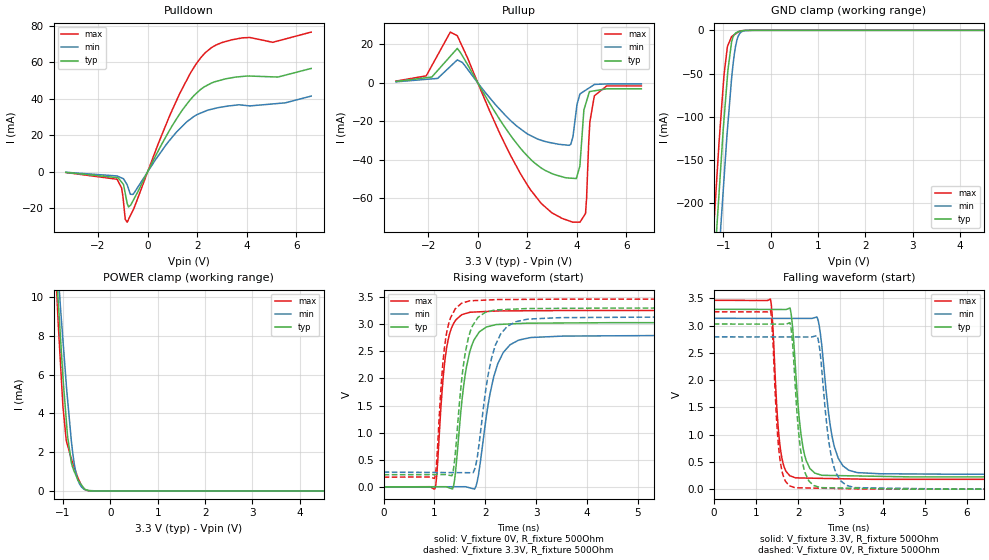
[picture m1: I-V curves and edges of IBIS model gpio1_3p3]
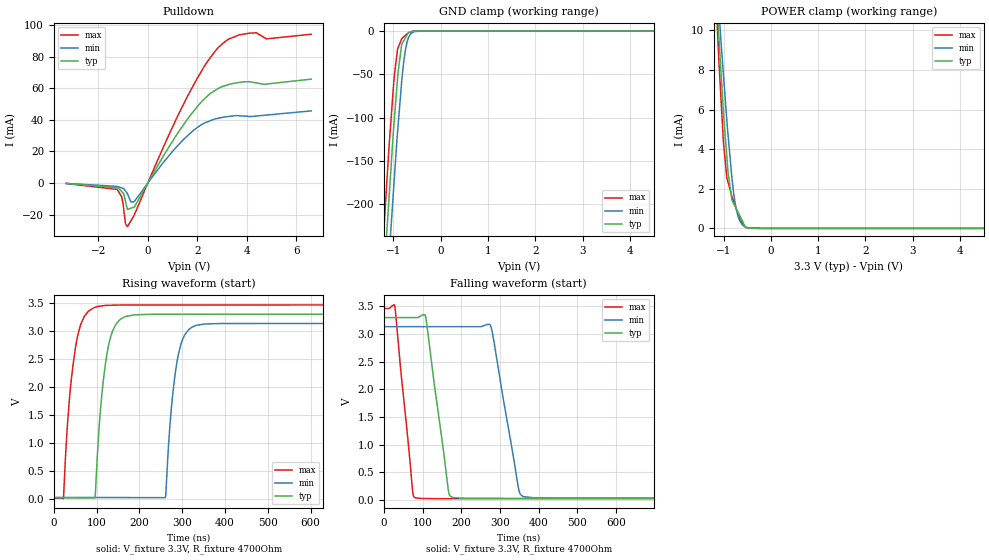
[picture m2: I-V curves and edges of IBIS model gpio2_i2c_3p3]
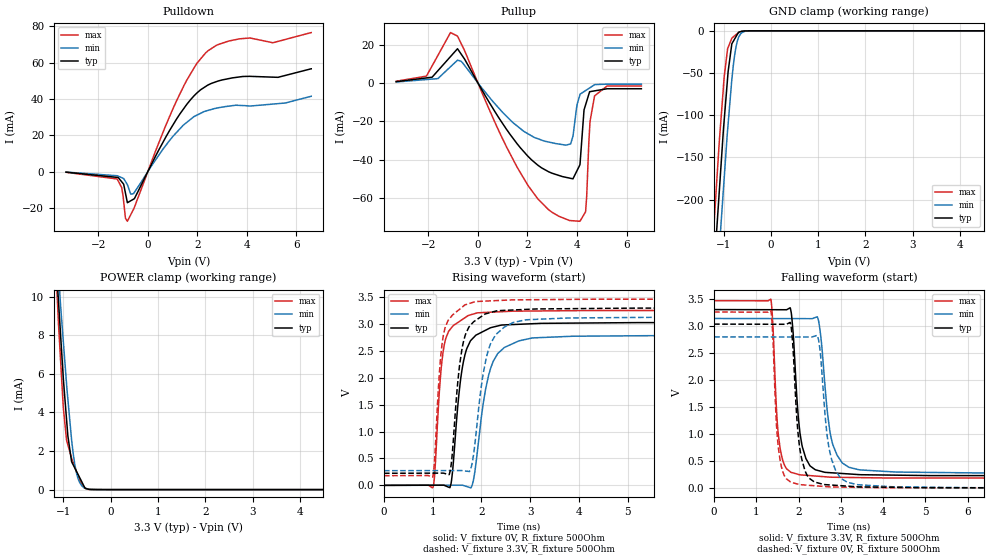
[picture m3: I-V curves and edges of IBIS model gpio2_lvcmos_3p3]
| Texas Instruments Incorporated
| CDCI6214
| Marketing part#   Digital Voltage Range   Package-type   #pins
| CDCI6214   1.71V - 3.465V   QFN   24
[IBIS Ver]   5.0
[File name]   cdci6214.ibs
[File Rev]   1.0
[Date]   10/26/2018
[Source]
| Texas Instruments Incorporated.
| Online Design Tools
| 12500 TI Blvd
| Dallas, TX -75243
[Notes]   Revision History:
| Rev 1.1: 10/26/2018
| - Pin1 and 2 name updated.
| Rev 1.0: 08/24/2017
| - Initial version of the model
| - Model generated from simulations in SPECTRE
| - Model matched to SPICE simulation
| - C_comp although listed in numerical order of value are
|   obtained from varying PVT conditions. For PVT conditions for
|   each specific value refer the buffer description under
|   respective [Model]. IBIS model user is responsible for using
|   appropriate C_comp to simulate for Signal Integrity.
| - Notes regarding combined Non-monotonicity of various models
|   have been reviewed and considered minor and can be ignored.
[Disclaimer]
| This model is designed as an aid for customers of Texas Instruments.
| TI and its licensors and suppliers make no warranties, either expressed
| or implied, with respect to this  model, including the warranties of
| merchantability or fitness for a particular purpose. The model is
| provided solely on an "as is" basis. The entire risk as to its quality
| and performance is with the customer.
[Copyright]
(C) Copyright 2017 Texas Instruments Incorporated.All rights reserved.
|   CDCI6214
[Component]   CDCI6214
[Manufacturer]   TI
[Package]   |24 QFN
|   typ   min   max
R_pkg   0.08328ohm   0.00805ohm   0.12644ohm
L_pkg   0.9771nH   0.25585nH   1.39654nH
C_pkg   0.1809pF   0.13118pF   0.62699pF
[Pin]   signal_name   model_name   R_pin   L_pin   C_pin
1   XOUT/FB   input1   0.00805ohm   0.25585nH   0.62699pF
2   XIN/FB   input2   0.08466ohm   0.93051nH   0.14630pF
3   VDD_REF   power   0.04341ohm   0.67199nH   0.16682pF
4   REF_SEL   input3   0.08490ohm   0.93218nH   0.14358pF
5   REFP   refp   0.08517ohm   0.93587nH   0.14543pF
6   REFN   refn   0.08525ohm   0.94279nH   0.13118pF
7   Y0   output   0.09517ohm   1.04961nH   0.13714pF
8   RESETN/SYNC   gpio1   0.08356ohm   0.91705nH   0.14348pF
9   Y4N   diff_out   0.08217ohm   0.90083nH   0.14310pF
10   Y4P   diff_out   0.09011ohm   0.98297nH   0.14845pF
11   OE/GPIO4   gpio1   0.08464ohm   0.92609nH   0.14498pF
12   SCL/GPIO3   input4   0.10102ohm   1.10915nH   0.14502pF
13   Y3N   diff_out   0.11209ohm   1.23284nH   0.15766pF
14   Y3P   diff_out   0.10303ohm   1.12457nH   0.16392pF
15   VDDO_34   power   0.03522ohm   0.70101nH   0.22084pF
16   VDDO_12   power   0.05257ohm   0.81073nH   0.20015pF
17   Y2N   diff_out   0.10909ohm   1.19284nH   0.16931pF
18   Y2P   diff_out   0.12644ohm   1.39654nH   0.16716pF
19   SDA/GPIO2   gpio2   0.05815ohm   0.96344nH   0.18512pF
20   STATUS/GPIO1   gpio1   0.10342ohm   1.13184nH   0.16054pF
21   Y1N   diff_out   0.10724ohm   1.17298nH   0.16355pF
22   Y1P   diff_out   0.10246ohm   1.12101nH   0.15895pF
23   EEPROMSEL   input3   0.10472ohm   1.14805nH   0.17052pF
24   VDD_VCO   power   0.05614ohm   0.89989nH   0.20226pF
[Diff Pin]   inv_pin   vdiff   tdelay_typ  tdelay_min  tdelay_max
5   6   200mV   NA   NA   NA
10   9   NA   NA   NA   NA
14   13   NA   NA   NA   NA
18   17   NA   NA   NA   NA
22   21   NA   NA   NA   NA
|   Model Selectors
[Model Selector] gpio1
gpio1_1p8   1.8V   I/O
gpio1_2p5   2.5V   I/O
gpio1_3p3   3.3V   I/O
[Model Selector] gpio2
gpio2_i2c_1p8   1.8V   I/O_open_drain
gpio2_i2c_2p5   2.5V   I/O_open_drain
gpio2_i2c_3p3   3.3V   I/O_open_drain
gpio2_lvcmos_1p8  1.8V   I/O
gpio2_lvcmos_2p5  2.5V   I/O
gpio2_lvcmos_3p3  3.3V   I/O
[Model Selector] input1
input1_1p8   1.8V   Input
input1_2p5   2.5V   Input
input1_3p3   3.3V   Input
[Model Selector] input2
input2_1p8   1.8V   Input
input2_2p5   2.5V   Input
input2_3p3   3.3V   Input
[Model Selector] input3
input3_1p8   1.8V   Input
input3_2p5   2.5V   Input
input3_3p3   3.3V   Input
[Model Selector] input4
input4_1p8   1.8V   Input
input4_2p5   2.5V   Input
input4_3p3   3.3V   Input
[Model Selector] output
output_fast_1p8   1.8V   3-state
output_fast_2p5   2.5V   3-state
output_fast_3p3   3.3V   3-state
output_slow_1p8   1.8V   3-state
output_slow_2p5   2.5V   3-state
output_slow_3p3   3.3V   3-state
[Model Selector] refn
refn_1p8   1.8V   Input
refn_2p5   2.5V   Input
refn_3p3   3.3V   Input
[Model Selector] refp
refp_1p8   1.8V   Input
refp_2p5   2.5V   Input
refp_3p3   3.3V   Input
[Model Selector] diff_out
cml_1p8   1.8V   3-state
cml_2p5   2.5V   3-state
cml_3p3   3.3V   3-state
hcsl_1p8   1.8V   Open_source
hcsl_2p5   2.5V   Open_source
hcsl_3p3   3.3V   Open_source
lvds_1p8   1.8V   3-state
lvds_2p5   2.5V   3-state
lvds_3p3   3.3V   3-state
lvpecl_1p8   1.8V   3-state
lvpecl_2p5   2.5V   3-state
lvpecl_3p3   3.3V   3-state
| Models and submodels in the file (45): gpio1_1p8 (I/O), gpio1_2p5 (I/O), gpio1_3p3 (I/O), gpio2_i2c_1p8 (I/O_open_drain), gpio2_i2c_2p5 (I/O_open_drain), gpio2_i2c_3p3 (I/O_open_drain), gpio2_lvcmos_1p8 (I/O), gpio2_lvcmos_2p5 (I/O), gpio2_lvcmos_3p3 (I/O), input1_1p8 (Input), input1_2p5 (Input), input1_3p3 (Input), input2_1p8 (Input), input2_2p5 (Input), input2_3p3 (Input), input3_1p8 (Input), input3_2p5 (Input), input3_3p3 (Input), input4_1p8 (Input), input4_2p5 (Input), input4_3p3 (Input), output_fast_1p8 (3-state), output_fast_2p5 (3-state), output_fast_3p3 (3-state), output_slow_1p8 (3-state), output_slow_2p5 (3-state), output_slow_3p3 (3-state), refn_1p8 (Input), refn_2p5 (Input), refn_3p3 (Input), refp_1p8 (Input), refp_2p5 (Input), refp_3p3 (Input), cml_1p8 (3-state), cml_2p5 (3-state), cml_3p3 (3-state), hcsl_1p8 (Open_source), hcsl_2p5 (Open_source), hcsl_3p3 (Open_source), lvds_1p8 (3-state), lvds_2p5 (3-state), lvds_3p3 (3-state), lvpecl_1p8 (3-state), lvpecl_2p5 (3-state), lvpecl_3p3 (3-state)
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|   gpio1_3p3 Model
[Model]   gpio1_3p3
Model_type   I/O
Polarity   Non-Inverting
Enable   Active-High
Vinl = 0.66
Vinh = 2.64
Vmeas = 1.65
Vref = 0
Cref = 2pF
Rref = 100000
|   typ   min   max
C_comp   1.218E-12   1.178E-12   1.263E-12
|  Where Nom  PVT is Nominal Process, 3.3V,   32C
|   Fast PVT is Strong Process,  3.465V, -35C
|   Slow PVT is Weak Process,   3.135V,  110C
[Model spec]
|subparameter
Vinl   0.66   0.627   0.693
Vinh   2.64   2.508   2.772
[Voltage Range]   3.3   3.135   3.465
|Junction Temperature
[Temperature Range]   32   110   -35
[Pullup Reference]   3.3   3.135   3.465
[Pulldown Reference]   0   0   0
[Power Clamp Reference]   3.3   3.135   3.465
[GND Clamp Reference]   0   0   0
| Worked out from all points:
|   slope of the pulldown table from 0 to 0.495 V, typ, clamps not added: 37.4 ohm
|   slope of the pullup table from 0 to 0.495 V, typ, clamps not added: 45.2 ohm
|   GND clamp passes 1 mA (typ) near -0.64 V on its own axis
|   POWER clamp passes 1 mA (typ) near -0.76 V on its own axis
|   falling waveform, V_fixture 3.3V, R_fixture 500Ohm: 20-80 % time 203ps typ, 269ps min, 151ps max; typ from 3.3 V to 0.225 V
|   rising waveform, V_fixture 0V, R_fixture 500Ohm: 20-80 % time 232ps typ, 316ps min, 172ps max; typ from 0 V to 3.03 V
|   rising waveform, V_fixture 3.3V, R_fixture 500Ohm: 20-80 % time 222ps typ, 297ps min, 167ps max; typ from 0.225 V to 3.3 V
|   falling waveform, V_fixture 0V, R_fixture 500Ohm: 20-80 % time 190ps typ, 244ps min, 144ps max; typ from 3.03 V to 0 V
[Pulldown]
|   Voltage   I(typ)   I(min)   I(max)
-3.3V     -281.2uA   -217.7uA   -339.4uA
-1.233V   -3.154mA   -2.235mA   -4.033mA
-1.053V   -5.544mA   -3.289mA   -8.714mA
-901.2mV  -11.85mA   -5.349mA   -25.93mA
-823.9mV  -17.27mA   -7.081mA   -27.52mA
-696.8mV  -18.36mA   -12.26mA   -24.01mA
-594.8mV  -15.96mA   -12.35mA   -21.19mA
1.294V    31.68mA    23.5mA     42.79mA
2.327V    46.8mA     33.2mA     65.19mA
3.412V    51.51mA    36.27mA    72.28mA
5.047V    51.96mA    37.15mA    70.86mA
6.6V      56.57mA    41.45mA    76.45mA
[GND Clamp]
|   Voltage   I(typ)   I(min)   I(max)
-3.3V     -2.319A    -2.382A    -2.268A
-1.236V   -318.8mA   -389.8mA   -259.2mA
-1.147V   -237.4mA   -310.6mA   -180.6mA
-1.055V   -160.4mA   -229.5mA   -104.5mA
-983.3mV  -102.7mA   -171.4mA   -51.26mA
-901.3mV  -45.9mA    -107.9mA   -17.34mA
-824.1mV  -13.56mA   -55.78mA   -7.292mA
-794.8mV  -8.05mA    -40.07mA   -6.183mA
-740.3mV  -3.37mA    -18.49mA   -4.155mA
-683.5mV  -1.418mA   -6.673mA   -2.04mA
-350.3mV  -1.174uA   -4.631uA   -305.6nA
6.6V      0A         0A         0A
[Pullup]
|   Voltage   I(typ)   I(min)   I(max)
-3.3V     687.4uA    501.9uA    887.3uA
-2.078V   2.634mA    1.794mA    3.583mA
-1.106V   13.78mA    8.472mA    26.32mA
-823.9mV  17.86mA    11.9mA     24.44mA
2.04V     -38.47mA   -26.81mA   -53.83mA
3.836V    -49.58mA   -28.22mA   -72.36mA
4.119V    -43.28mA   -5.949mA   -72.34mA
4.281V    -14.15mA   -4.441mA   -69.18mA
4.348V    -11.31mA   -3.883mA   -67.84mA
4.524V    -4.542mA   -2.406mA   -20.15mA
4.706V    -4.156mA   -879.2uA   -6.74mA
6.6V      -3.112mA   -581uA     -1.625mA
[POWER Clamp]
|   Voltage   I(typ)   I(min)   I(max)
-3.3V     111.2mA    95.93mA    136.6mA
-1.136V   11.16mA    12.47mA    10.45mA
-1.1V     9.757mA    11.16mA    8.588mA
-1.053V   7.912mA    9.452mA    6.571mA
-1.001V   5.871mA    7.768mA    4.346mA
-930.9mV  3.658mA    5.495mA    2.593mA
-904.3mV  2.832mA    4.732mA    2.358mA
-824.1mV  1.459mA    2.585mA    1.648mA
-727.5mV  803uA      934.1uA    973.7uA
-653.2mV  451.6uA    369.8uA    500.4uA
-542.3mV  82.36uA    69.06uA    85.37uA
6.6V      0A         0A         0A
[Ramp]
R_load = 500
|   typ   min   max
dV/dt_r   1.81838/2.29343e-10   1.67671/3.14244e-10   1.95286/1.70968e-10
dV/dt_f   1.84525/2.00647e-10   1.71729/2.67311e-10   1.97107/1.50595e-10
[Falling Waveform]
V_fixture = 3.3V
V_fixture_min = 3.135V
V_fixture_max = 3.465V
R_fixture = 500Ohm
C_fixture = 0F
|   Time   V(typ)   V(min)   V(max)
0s        3.3V       3.135V     3.465V
1.342ns   3.298V     3.133V     3.488V
1.584ns   3.298V     3.133V     709.5mV
1.812ns   3.307V     3.133V     243.2mV
1.94ns    2.172V     3.133V     207.2mV
2.278ns   379.4mV    3.132V     202.1mV
2.477ns   274.7mV    3.085V     199.1mV
2.86ns    250.2mV    771.8mV    193.5mV
3.396ns   242.7mV    304.4mV    185.6mV
25ns      224.6mV    272.9mV    179.9mV
[Rising Waveform]
V_fixture = 0V
V_fixture_min = 0V
V_fixture_max = 0V
R_fixture = 500Ohm
C_fixture = 0F
|   Time   V(typ)   V(min)   V(max)
0s        -402.5nV   -288.2nV   -1.368uV
1.01ns    2.656mV    1.881mV    -31.91mV
1.192ns   3.134mV    2.219mV    2.219V
1.356ns   -37.73mV   2.525mV    2.975V
1.574ns   1.861V     2.93mV     3.188V
1.7ns     2.509V     -18.83mV   3.222V
1.841ns   2.801V     98.92mV    3.228V
2.244ns   2.996V     2.269V     3.246V
2.893ns   3.02V      2.755V     3.25V
25ns      3.031V     2.795V     3.255V
[Rising Waveform]
V_fixture = 3.3V
V_fixture_min = 3.135V
V_fixture_max = 3.465V
R_fixture = 500Ohm
C_fixture = 0F
|   Time   V(typ)   V(min)   V(max)
0s        224.6mV    272.9mV    179.9mV
1.002ns   226.9mV    266.2mV    157.3mV
1.181ns   227.3mV    265mV      2.433V
1.342ns   206.6mV    263.9mV    3.167V
1.556ns   2.143V     262.5mV    3.394V
1.694ns   2.834V     261.6mV    3.433V
1.823ns   3.08V      448.2mV    3.438V
2.198ns   3.265V     2.615V     3.454V
2.837ns   3.289V     3.095V     3.459V
25ns      3.3V       3.135V     3.465V
[Falling Waveform]
|Gnd
V_fixture = 0V
V_fixture_min = 0V
V_fixture_max = 0V
R_fixture = 500Ohm
C_fixture = 0F
|   Time   V(typ)   V(min)   V(max)
0s        3.031V     2.795V     3.255V
1.342ns   3.029V     2.793V     3.277V
1.572ns   3.028V     2.793V     528.5mV
1.811ns   3.038V     2.793V     57.92mV
1.925ns   1.968V     2.793V     26.05mV
2.254ns   149.4mV    2.792V     21.24mV
2.472ns   41.97mV    2.751V     18.12mV
2.86ns    23.52mV    376.5mV    12.6mV
3.337ns   17.16mV    28.73mV    5.79mV
25ns      -291.6nV   86.34nV    -1.136uV
|   gpio2_i2c_3p3 Model
[Model]   gpio2_i2c_3p3
Model_type   I/O_open_drain
Polarity   Inverting
Enable   Active-High
Vinl = 0.66
Vinh = 2.64
Vmeas = 1.65
Vref = 3.3
Cref = 1pF
Rref = 4700
|   typ   min   max
C_comp   1.748E-12   1.672E-12   1.811E-12
|  Where Nom  PVT is Nominal Process, 3.3V,   32C
|   Fast PVT is Strong Process,  3.465V, -35C
|   Slow PVT is Weak Process,   3.135V,  110C
[Model spec]
|subparameter
Vinl   0.66   0.627   0.693
Vinh   2.64   2.508   2.772
[Voltage Range]   3.3   3.135   3.465
|Junction Temperature
[Temperature Range]   32   110   -35
[Pullup Reference]   3.3   3.135   3.465
[Pulldown Reference]   -0   0   0
[Power Clamp Reference]   3.3   3.135   3.465
[GND Clamp Reference]   0   0   0
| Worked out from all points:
|   slope of the pulldown table from 0 to 0.495 V, typ, clamps not added: 36.6 ohm
|   GND clamp passes 1 mA (typ) near -0.64 V on its own axis
|   POWER clamp passes 1 mA (typ) near -0.73 V on its own axis
|   falling waveform, V_fixture 3.3V, R_fixture 4700Ohm: 20-80 % time 37.3ns typ, 45ns min, 29.2ns max; typ from 3.3 V to 0.025 V
|   rising waveform, V_fixture 3.3V, R_fixture 4700Ohm: 20-80 % time 24.4ns typ, 23.6ns min, 25.3ns max; typ from 0.025 V to 3.3 V
[Pulldown]
|   Voltage   I(typ)   I(min)   I(max)
-3.3V     -271.3uA   -200.8uA   -336.9uA
-1.234V   -3.077mA   -2.137mA   -4.024mA
-1.054V   -5.398mA   -3.111mA   -8.712mA
-901.7mV  -11.53mA   -5.025mA   -25.76mA
-824.4mV  -16.75mA   -6.638mA   -27.6mA
-562.7mV  -15.26mA   -11.93mA   -20.76mA
1.435V    36.74mA    27.52mA    49.7mA
2.216V    52.21mA    37.42mA    72.18mA
2.847V    60.01mA    41.05mA    85.86mA
4.119V    64.22mA    42.09mA    94.98mA
4.791V    62.71mA    43.06mA    91.35mA
6.6V      65.84mA    45.73mA    94.28mA
[GND Clamp]
|   Voltage   I(typ)   I(min)   I(max)
-3.3V     -2.319A    -2.383A    -2.268A
-1.251V   -332.8mA   -408mA     -272.7mA
-1.148V   -239.4mA   -314.9mA   -182.6mA
-1.056V   -161.7mA   -230.8mA   -106.1mA
-985.8mV  -105.5mA   -174.3mA   -54.27mA
-902.9mV  -48.28mA   -110.2mA   -19.61mA
-824.7mV  -15.34mA   -57.67mA   -8.718mA
-793.4mV  -12.33mA   -41.07mA   -7.201mA
-737.9mV  -7.013mA   -19.49mA   -4.561mA
-682.2mV  -1.725mA   -7.797mA   -2.276mA
-339mV    -1.939uA   -4.787uA   -28.93uA
6.6V      0A         0A         0A
[POWER Clamp]
|   Voltage   I(typ)   I(min)   I(max)
-3.3V     110.9mA    95.66mA    136.2mA
-1.137V   11.14mA    12.45mA    10.43mA
-1.1V     9.694mA    11.11mA    8.517mA
-1.054V   7.896mA    9.439mA    6.554mA
-1.001V   5.816mA    7.724mA    4.293mA
-930.4mV  3.619mA    5.455mA    2.558mA
-903.9mV  2.799mA    4.702mA    2.327mA
-824.7mV  1.449mA    2.586mA    1.636mA
-759.7mV  1.135mA    1.347mA    1.188mA
-693.4mV  813.9uA    612.2uA    731.8uA
-517.5mV  60.13uA    50.11uA    39.96uA
6.6V      0A         0A         0A
[Ramp]
R_load = 4700
|   typ   min   max
dV/dt_r   1.96507/2.43683e-08   1.86267/2.36459e-08   2.06717/2.52368e-08
dV/dt_f   1.96507/3.72443e-08   1.86268/4.49716e-08   2.06717/2.91919e-08
[Falling Waveform]
V_fixture = 3.3V
V_fixture_min = 3.135V
V_fixture_max = 3.465V
R_fixture = 4700Ohm
C_fixture = 0F
|   Time   V(typ)   V(min)   V(max)
0s        3.3V       3.135V     3.465V
28.07ns   3.3V       3.135V     3.507V
74.03ns   3.299V     3.135V     160mV
80.31ns   3.299V     3.135V     37.47mV
107.6ns   3.316V     3.135V     22.37mV
165.9ns   197.7mV    3.134V     20.18mV
175.9ns   46.67mV    3.134V     20.18mV
275.1ns   25.72mV    3.164V     20.13mV
359.5ns   25.64mV    62.77mV    20.09mV
1.2us     24.84mV    30.47mV    19.68mV
[Rising Waveform]
V_fixture = 3.3V
V_fixture_min = 3.135V
V_fixture_max = 3.465V
R_fixture = 4700Ohm
C_fixture = 0F
|   Time   V(typ)   V(min)   V(max)
0s        24.84mV    30.47mV    19.68mV
22.39ns   23.5mV     30.08mV    14.81mV
55.6ns    21.51mV    29.51mV    2.908V
93.84ns   19.22mV    28.84mV    3.416V
124.3ns   2.598V     28.31mV    3.457V
167.3ns   3.257V     27.57mV    3.464V
260.5ns   3.299V     25.95mV    3.464V
288.5ns   3.299V     2.481V     3.464V
330.8ns   3.299V     3.095V     3.464V
1.2us     3.3V       3.135V     3.465V
|   gpio2_lvcmos_3p3 Model
[Model]   gpio2_lvcmos_3p3
Model_type   I/O
Polarity   Non-Inverting
Enable   Active-High
Vinl = 0.66
Vinh = 2.64
Vmeas = 1.65
Vref = 0
Cref = 1pF
Rref = 100000
|   typ   min   max
C_comp   1.748E-12   1.672E-12   1.811E-12
|  Where Nom  PVT is Nominal Process, 3.3V,   32C
|   Fast PVT is Strong Process,  3.465V, -35C
|   Slow PVT is Weak Process,   3.135V,  110C
[Model spec]
|subparameter
Vinl   0.66   0.627   0.693
Vinh   2.64   2.508   2.772
[Voltage Range]   3.3   3.135   3.465
|Junction Temperature
[Temperature Range]   32   110   -35
[Pullup Reference]   3.3   3.135   3.465
[Pulldown Reference]   0   0   0
[Power Clamp Reference]   3.3   3.135   3.465
[GND Clamp Reference]   0   0   0
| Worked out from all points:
|   slope of the pulldown table from 0 to 0.495 V, typ, clamps not added: 37.5 ohm
|   slope of the pullup table from 0 to 0.495 V, typ, clamps not added: 45.2 ohm
|   GND clamp passes 1 mA (typ) near -0.64 V on its own axis
|   POWER clamp passes 1 mA (typ) near -0.73 V on its own axis
|   falling waveform, V_fixture 3.3V, R_fixture 500Ohm: 20-80 % time 182ps typ, 238ps min, 140ps max; typ from 3.3 V to 0.225 V
|   rising waveform, V_fixture 0V, R_fixture 500Ohm: 20-80 % time 221ps typ, 304ps min, 166ps max; typ from 0 V to 3.03 V
|   rising waveform, V_fixture 3.3V, R_fixture 500Ohm: 20-80 % time 211ps typ, 284ps min, 161ps max; typ from 0.225 V to 3.3 V
|   falling waveform, V_fixture 0V, R_fixture 500Ohm: 20-80 % time 176ps typ, 228ps min, 135ps max; typ from 3.03 V to 0 V
[Pulldown]
|   Voltage   I(typ)   I(min)   I(max)
-3.3V     -282uA     -218.3uA   -340.4uA
-1.238V   -3.145mA   -2.234mA   -4.022mA
-1.057V   -5.516mA   -3.29mA    -8.642mA
-902.6mV  -11.78mA   -5.37mA    -25.59mA
-824.4mV  -17.06mA   -7.121mA   -27.29mA
-694.4mV  -16.03mA   -12.17mA   -23.79mA
-585.5mV  -15.18mA   -12.14mA   -20.87mA
1.153V    28.75mA    21.44mA    38.72mA
2.331V    46.78mA    33.28mA    65.24mA
3.695V    52.07mA    36.44mA    73.01mA
5.053V    51.96mA    37.17mA    70.88mA
6.6V      56.58mA    41.46mA    76.48mA
[GND Clamp]
|   Voltage   I(typ)   I(min)   I(max)
-3.3V     -2.319A    -2.383A    -2.268A
-1.251V   -332.8mA   -408mA     -272.7mA
-1.148V   -239.4mA   -314.9mA   -182.6mA
-1.056V   -161.7mA   -230.8mA   -106.1mA
-985.8mV  -105.5mA   -174.3mA   -54.27mA
-902.9mV  -48.28mA   -110.2mA   -19.61mA
-824.7mV  -15.34mA   -57.67mA   -8.718mA
-793.4mV  -12.33mA   -41.07mA   -7.201mA
-737.9mV  -7.013mA   -19.49mA   -4.561mA
-682.2mV  -1.725mA   -7.797mA   -2.276mA
-339mV    -1.939uA   -4.787uA   -28.93uA
6.6V      0A         0A         0A
[Pullup]
|   Voltage   I(typ)   I(min)   I(max)
-3.3V     687.3uA    501.9uA    887.3uA
-2.078V   2.636mA    1.793mA    3.587mA
-1.107V   13.79mA    8.471mA    26.31mA
-824.4mV  17.87mA    11.9mA     24.45mA
1.153V    -24.17mA   -17.37mA   -33.34mA
2.672V    -45.04mA   -30.29mA   -63.82mA
3.743V    -49.79mA   -31.82mA   -71.84mA
4.119V    -42.73mA   -6.156mA   -72.22mA
4.348V    -11.39mA   -3.965mA   -67.2mA
4.527V    -4.524mA   -2.463mA   -20.06mA
4.711V    -4.124mA   -928uA     -6.737mA
6.6V      -3.021mA   -617.7uA   -1.587mA
[POWER Clamp]
|   Voltage   I(typ)   I(min)   I(max)
-3.3V     110.9mA    95.66mA    136.2mA
-1.137V   11.14mA    12.45mA    10.43mA
-1.1V     9.694mA    11.11mA    8.517mA
-1.054V   7.896mA    9.439mA    6.554mA
-1.001V   5.816mA    7.724mA    4.293mA
-930.4mV  3.619mA    5.455mA    2.558mA
-903.9mV  2.799mA    4.702mA    2.327mA
-824.7mV  1.449mA    2.586mA    1.636mA
-759.7mV  1.135mA    1.347mA    1.188mA
-693.4mV  813.9uA    612.2uA    731.8uA
-517.5mV  60.13uA    50.11uA    39.96uA
6.6V      0A         0A         0A
[Ramp]
R_load = 500
|   typ   min   max
dV/dt_r   1.81837/2.20865e-10   1.67668/3.03168e-10   1.95286/1.65864e-10
dV/dt_f   1.84523/1.80297e-10   1.71726/2.38078e-10   1.97106/1.37954e-10
[Falling Waveform]
V_fixture = 3.3V
V_fixture_min = 3.135V
V_fixture_max = 3.465V
R_fixture = 500Ohm
C_fixture = 0F
|   Time   V(typ)   V(min)   V(max)
0s        3.3V       3.135V     3.465V
1.341ns   3.298V     3.133V     3.493V
1.488ns   3.297V     3.133V     1.298V
1.558ns   3.297V     3.133V     755.7mV
1.824ns   3.248V     3.133V     286.5mV
2.019ns   1.101V     3.132V     243.5mV
2.446ns   324.1mV    3.159V     216.5mV
2.794ns   278.2mV    843mV      196.8mV
3.429ns   245.1mV    334.5mV    189.7mV
25ns      224.6mV    272.9mV    179.9mV
[Rising Waveform]
V_fixture = 0V
V_fixture_min = 0V
V_fixture_max = 0V
R_fixture = 500Ohm
C_fixture = 0F
|   Time   V(typ)   V(min)   V(max)
0s        -761.5nV   -858.6nV   -28.61nV
1.008ns   2.781mV    1.937mV    -34.53mV
1.188ns   3.277mV    2.283mV    2.3V
1.354ns   -41.05mV   2.602mV    2.898V
1.624ns   2.273V     -330.5uV   3.096V
1.789ns   2.703V     -41.08mV   3.176V
1.909ns   2.805V     574.7mV    3.208V
2.246ns   2.946V     2.314V     3.224V
3.059ns   3.008V     2.744V     3.244V
25ns      3.031V     2.794V     3.255V
[Rising Waveform]
V_fixture = 3.3V
V_fixture_min = 3.135V
V_fixture_max = 3.465V
R_fixture = 500Ohm
C_fixture = 0F
|   Time   V(typ)   V(min)   V(max)
0s        224.6mV    272.9mV    179.9mV
998.3ps   227mV      274.3mV    150.9mV
1.178ns   227.5mV    274.5mV    2.522V
1.341ns   205.3mV    274.7mV    3.096V
1.601ns   2.54V      274.2mV    3.314V
1.769ns   2.972V     279.5mV    3.389V
1.869ns   3.062V     799.3mV    3.418V
2.186ns   3.216V     2.631V     3.433V
2.919ns   3.274V     3.081V     3.453V
25ns      3.3V       3.135V     3.465V
[Falling Waveform]
|Gnd
V_fixture = 0V
V_fixture_min = 0V
V_fixture_max = 0V
R_fixture = 500Ohm
C_fixture = 0F
|   Time   V(typ)   V(min)   V(max)
0s        3.031V     2.794V     3.255V
1.341ns   3.028V     2.793V     3.282V
1.478ns   3.028V     2.793V     1.144V
1.558ns   3.028V     2.793V     535.3mV
1.824ns   2.972V     2.792V     101.8mV
2.019ns   775.5mV    2.792V     61.32mV
2.446ns   93.41mV    2.814V     34.92mV
2.766ns   52.54mV    566.8mV    16.42mV
3.389ns   19.74mV    59.33mV    9.73mV
25ns      -1.099uV   -686.7nV   74.01nV
